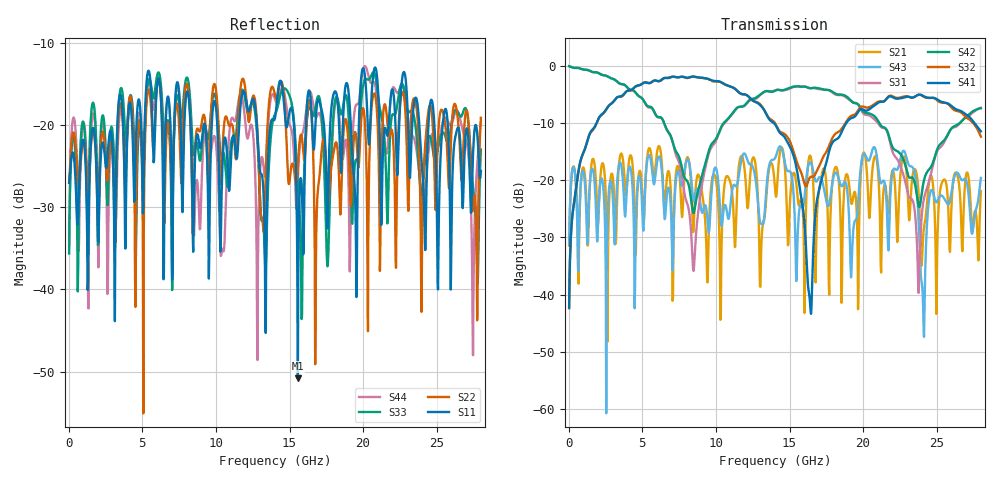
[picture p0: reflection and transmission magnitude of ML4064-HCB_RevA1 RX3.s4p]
! TOUCHSTONE file generated by CST DESIGN STUDIO
! Date and time: Wed Aug 26 10:42:10 2020
! Project name:  Project name: C:\Users\Simulation2\Temp\DE66\Untitled_0.cst
! Tree item: Tasks\SPara1\S-Parameters
# GHz S MA R 50
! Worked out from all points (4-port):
!   1000 points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, 28 MHz to 28 GHz, reference 50 ohm
!   strongest paths, dB at 28 MHz, 7.028 GHz, 14.03 GHz, 21.03 GHz, 28 GHz:
!     S41: -42.3, -1.9, -10.3, -6.4, -11.5
!     S32: -42.4, -1.9, -10.1, -6.3, -12.4
!     S42: -0.1, -13.0, -4.4, -9.7, -7.4
!     S31: -0.1, -13.0, -4.3, -10.1, -7.4
!     S43: -31.0, -32.8, -16.1, -17.8, -19.6
!     S21: -31.4, -31.4, -21.8, -19.0, -21.9
!   lowest |S11| = -50.8 dB at 15.57 GHz (marker M1), VSWR 1.01, Z = 50 + j0.287 ohm
!   |S11| at or under -10 dB: start of sweep to end of sweep
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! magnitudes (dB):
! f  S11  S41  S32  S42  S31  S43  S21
! 28 MHz  -27.0  -42.3  -42.4  -0.1  -0.1  -31.0  -31.4
! 8.484 GHz  -32.4  -1.9  -1.9  -25.7  -35.9  -23.6  -28.5
! 15.57 GHz  -50.8  -19.2  -17.3  -3.6  -3.6  -28.8  -23.5
! 16.38 GHz  -16.0  -41.0  -19.6  -3.9  -3.9  -16.9  -15.7
! 17.86 GHz  -17.6  -13.7  -12.9  -4.5  -4.6  -21.3  -21.8
! 23.77 GHz  -18.8  -5.1  -5.0  -24.5  -39.7  -27.3  -22.3
! 28 GHz  -25.6  -11.5  -12.4  -7.4  -7.4  -19.6  -21.9
